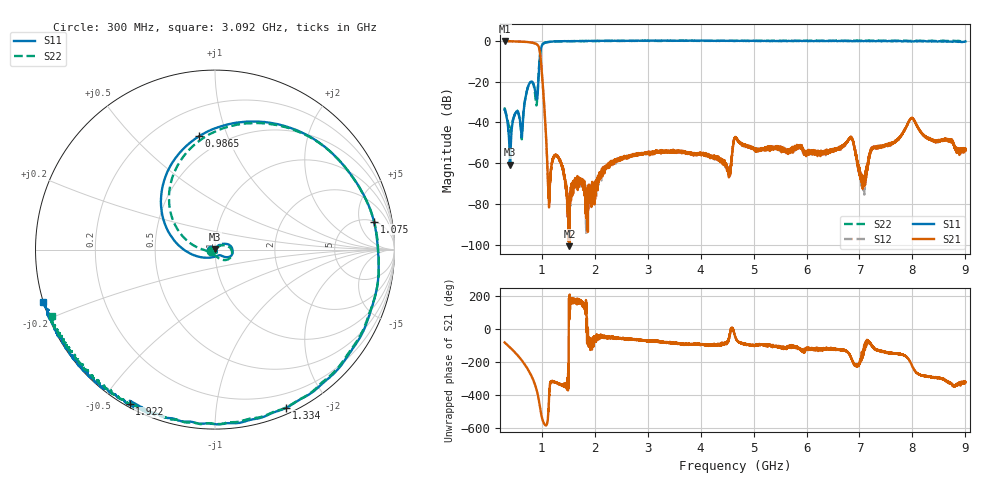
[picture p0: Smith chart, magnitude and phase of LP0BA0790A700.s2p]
!Agilent Technologies,E8358A,US41080443,A.07.50.56
!Agilent E8358A: A.07.50.56
!Date: Monday, December 14, 2015 12:30:56
!Correction: S11(Full 2 Port(1,2))
!S21(Full 2 Port(1,2))
!S12(Full 2 Port(1,2))
!S22(Full 2 Port(1,2))
!S2P File: Measurements: S11, S21, S12, S22:
# Hz S  dB  R 50
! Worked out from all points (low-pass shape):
!   6401 points, 300 MHz to 9 GHz, reference 50 ohm
!   highest |S21| = -0.20 dB at 300 MHz (marker M1); lowest = -100.5 dB at 1.523 GHz (marker M2)
!   |S21| within 3 dB of the highest: start of sweep to 946.7 MHz
!   lowest |S11| = -60.7 dB at 406 MHz (marker M3), VSWR 1.00, Z = 50.1 + j0.0671 ohm
!   |S11| at or under -10 dB: start of sweep to 959.5 MHz
!   |S22| runs from -48.3 to 0.1 dB; largest |S21 - S12| = 0.0076
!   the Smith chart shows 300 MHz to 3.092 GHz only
!   S11 on the Smith chart (normalised r, x): 300 MHz: 0.96, -0.01; 986.5 MHz: 0.37, +0.80; 1.075 GHz: 5.14, +8.34; 1.334 GHz: 0.06, -1.54; 1.922 GHz: 0.01, -0.59; 3.092 GHz: -0.00, -0.15
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3e8  -33.67 -172.5  -0.20 -81.4  -0.21 -81.2  -33.32 -164.2
4.060312e8  -60.65 46.2  -0.27 -112.9  -0.27 -112.7  -44.39 -119.1
6.085781e8  -43.29 -63.5  -0.46 176.5  -0.44 176.7  -43.40 -71.0
7.67625e8  -20.93 12.8  -0.80 100.4  -0.79 100.7  -21.00 2.5
8.858906e8  -26.05 -43.0  -1.46 11.4  -1.45 11.8  -28.78 -84.0
9.864844e8  -3.91 97.9  -10.34 -149.1  -10.32 -148.7  -3.67 90.4
1.074844e9  -0.92 10.0  -43.21 136.4  -43.15 136.1  -0.89 8.3
1.142812e9  -0.62 -20.0  -78.50 -44.1  -79.53 -52.0  -0.63 -20.7
1.334484e9  -0.29 -65.9  -58.25 27.9  -57.65 25.8  -0.32 -65.4
1.523438e9  -0.27 -91.8  -100.55 57.9  -80.87 127.1  -0.28 -91.2
1.750453e9  -0.25 -114.7  -68.68 161.3  -67.52 171.4  -0.21 -111.7
1.921734e9  -0.14 -118.9  -72.93 -76.7  -71.80 -85.0  -0.23 -118.1
3.092156e9  0.03 -163.0  -55.21 -67.5  -54.94 -67.8  -0.17 -157.8
3.200906e9  0.01 -164.7  -54.08 -75.8  -54.33 -73.3  -0.18 -160.3
4.529016e9  -0.11 -178.2  -65.59 -66.4  -63.60 -76.2  -0.12 -178.8
4.65e9  -0.11 -179.2  -47.36 -42.2  -47.41 -39.8  -0.15 179.6
6.100453e9  -0.12 157.6  -55.35 -123.7  -55.26 -123.8  -0.12 155.9
6.841312e9  -0.16 149.9  -47.44 -173.9  -47.05 -173.5  -0.03 152.3
7.066969e9  -0.20 149.3  -68.87 -147.2  -70.29 -150.8  0.02 152.6
7.550906e9  -0.13 150.7  -51.08 -147.3  -50.96 -140.3  -0.06 151.5
7.988625e9  -0.42 151.5  -37.89 140.4  -37.95 142.0  -0.16 148.9
9e9  -0.40 142.9  -53.70 36.4  -52.30 40.4  -0.18 132.3
